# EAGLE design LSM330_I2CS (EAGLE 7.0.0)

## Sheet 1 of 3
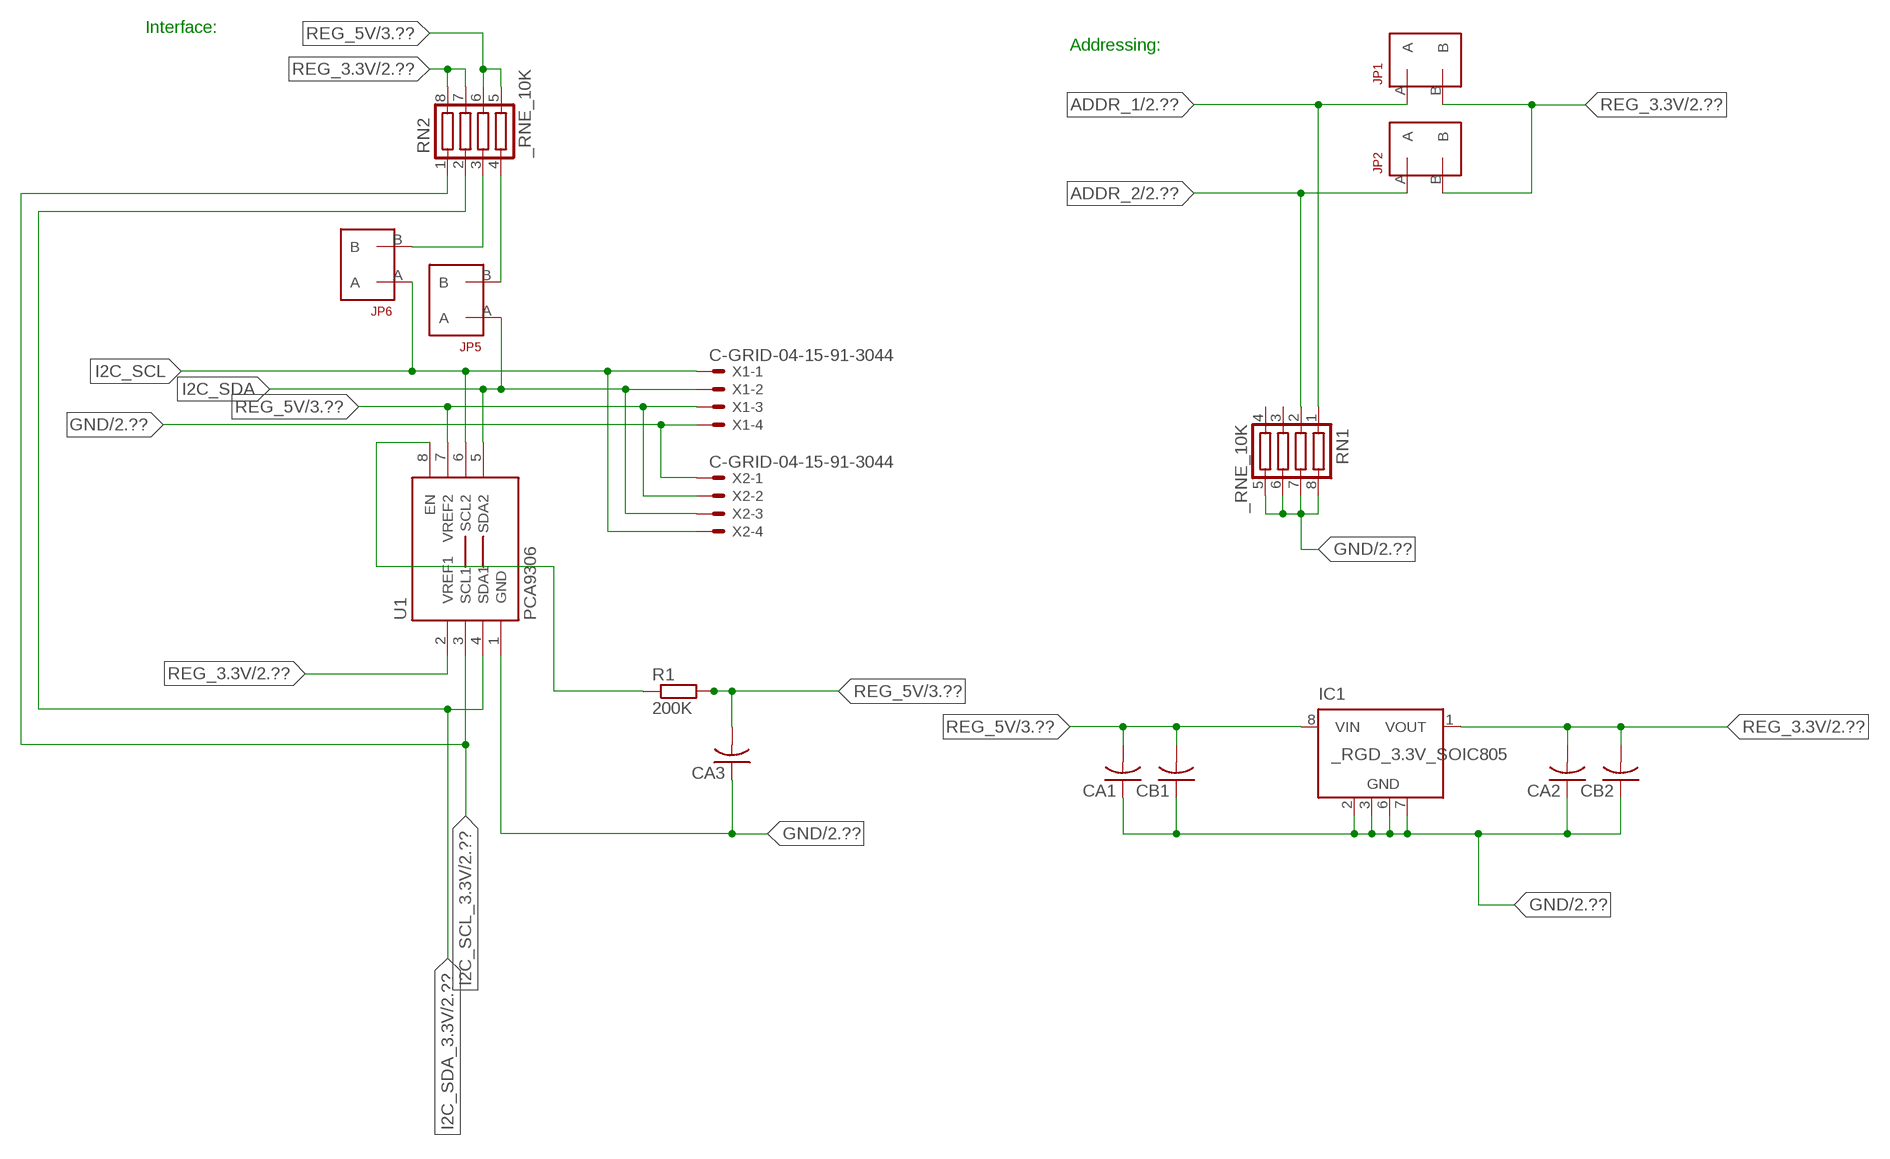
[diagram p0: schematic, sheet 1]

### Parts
CA1  CC1206KRX7R9BB104  [.1UF]
CA2  CC1206KRX7R9BB104  [.1UF]
CA3  CC1206KRX7R9BB104  [.1UF]
CB1  TMK316F106ZL-TC1206K  [TMK316F106ZL-T]
CB2  TMK316F106ZL-TC1206K  [TMK316F106ZL-T]
IC1  _RGD_3.3V_SOIC805  [_RGC_3.3V_SOIC8]
JP1  JUMPER_1X2_2MM  [JUMPER_1X2_2MM]
JP2  JUMPER_1X2_2MM  [JUMPER_1X2_2MM]
JP5  JUMPER_1X2_2MM  [JUMPER_1X2_2MM]
JP6  JUMPER_1X2_2MM  [JUMPER_1X2_2MM]
R1  200K  RESISTOR_SMT-0603  [R603]
RN1  _RNE_10K  [RNE]
RN2  _RNE_10K  [RNE]
U1  PCA9306  PCA9306_NCD  [PSOP-8]
X1  C-GRID-04-15-91-3044  [15-91-04]
X2  C-GRID-04-15-91-3044  [15-91-04]

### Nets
ADDR_1: JP1.A RN1.1 ; also sheet 2
ADDR_2: JP2.A RN1.2 ; also sheet 2
GND: CA1.1 CA2.1 CA3.1 CB1.1 CB2.1 IC1.2(GND) IC1.3(GND) IC1.6(GND) IC1.7(GND) RN1.5 RN1.6 RN1.7 RN1.8 U1.1(GND) X1.4 X2.1 ; also sheet 2,3
I2C_SCL: JP6.A U1.6(SCL2) X1.1 X2.4
I2C_SCL_3.3V: RN2.1 U1.3(SCL1) ; also sheet 2
I2C_SDA: JP5.A U1.5(SDA2) X1.2 X2.3
I2C_SDA_3.3V: RN2.2 U1.4(SDA1) ; also sheet 2
N$1: JP6.B RN2.3
N$2: JP5.B RN2.4
N$3: R1.1 U1.8(EN)
REG_3.3V: CA2.2 CB2.2 IC1.1(VOUT) JP1.B JP2.B RN2.7 RN2.8 U1.2(VREF1) ; also sheet 2
REG_5V: CA1.2 CA3.2 CB1.2 IC1.8(VIN) R1.2 RN2.5 RN2.6 U1.7(VREF2) X1.3 X2.2 ; also sheet 3
Unconnected: IC1.4(NC) IC1.5(NC) RN1.3 RN1.4

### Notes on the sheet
- Interface:
- Addressing:

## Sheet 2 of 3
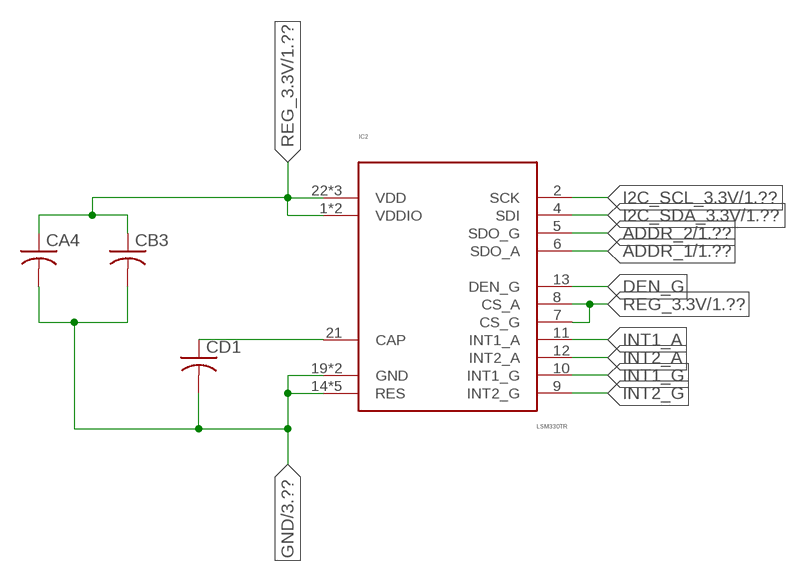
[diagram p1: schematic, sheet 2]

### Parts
CA4  CC1206KRX7R9BB104  [.1UF]
CB3  TMK316F106ZL-TC1206K  [TMK316F106ZL-T]
CD1  CC1206KRX7R9BB103C1206K  [CC1206KRX7R9BB103]
IC2  LSM330TR  LSM330  [LSM330]

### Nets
ADDR_1: IC2.6(SDO_A) ; also sheet 1
ADDR_2: IC2.5(SDO_G) ; also sheet 1
DEN_G: IC2.13(DEN_G)
GND: CA4.2 CB3.2 CD1.2 IC2.14(RES) IC2.15(RES) IC2.16(RES) IC2.17(RES) IC2.18(RES) IC2.19(GND) IC2.20(GND) ; also sheet 1,3
I2C_SCL_3.3V: IC2.2(SCK) ; also sheet 1
I2C_SDA_3.3V: IC2.4(SDI) ; also sheet 1
INT1_A: IC2.11(INT1_A)
INT1_G: IC2.10(INT1_G)
INT2_A: IC2.12(INT2_A)
INT2_G: IC2.9(INT2_G)
N$16: CD1.1 IC2.21(CAP)
REG_3.3V: CA4.1 CB3.1 IC2.1(VDDIO) IC2.3(VDDIO) IC2.7(CS_G) IC2.8(CS_A) IC2.22(VDD) IC2.23(VDD) IC2.24(VDD) ; also sheet 1

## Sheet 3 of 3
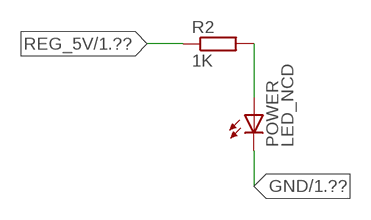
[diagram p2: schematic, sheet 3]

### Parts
POWER  LED_NCD  [CHIPLED_0603]
R2  1K  RESISTOR_SMT-0402  [R402]

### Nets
GND: POWER.C ; also sheet 1,2
N$4: POWER.A R2.2
REG_5V: R2.1 ; also sheet 1

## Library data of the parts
CA1-CA3 = NCD_ULTIMATE_LIBRARY:CC1206KRX7R9BB104: Capacitor CA .1uF 50V SMT C1206K CC1206KRX7R9BB104
CA4 = NCD_ULTIMATE_LIBRARY (2):CC1206KRX7R9BB104: Capacitor CA .1uF 50V SMT C1206K CC1206KRX7R9BB104
CB1 CB2 = NCD_ULTIMATE_LIBRARY:TMK316F106ZL-T: Capacitor CB 10uF SMT 1206 TMK316F106ZL-T
CB3 = NCD_ULTIMATE_LIBRARY (2):TMK316F106ZL-T: Capacitor CB 10uF SMT 1206 TMK316F106ZL-T
CD1 = NCD_ULTIMATE_LIBRARY (2):CC1206KRX7R9BB103: Capacitor CD .01uF SMT CC1206KRX7R9BB103 1206
IC1 = NCD_ULTIMATE_LIBRARY:_RGD_3.3V_SOIC8: Regulator Linear 3.3V Chip Positive VOLTAGE REGULATOR Digikey 497-1199-2-ND/L78L33ACD13TR
IC2 = NCD_ULTIMATE_KAMNA:LSM330
JP1 JP2 JP5 JP6 = NCD_ULTIMATE_CONNECTORS:JUMPER_1X2_2MM
POWER = NCD_ULTIMATE_LIBRARY:LED_NCD: LED Digikey 754-1132-2-ND/APT2012SRCPRV
R1 R2 = NCD_ULTIMATE_LIBRARY:RESISTOR_SMT: NCD Resistor
RN1 RN2 = NCD_ULTIMATE_LIBRARY:_RNE_10K: Resistor Array RNE SMT 10K x 4 Single Resistor Source: http://www.ctscorp.com/components/Datasheets/CTSChipArrayDs.pdf Digikey 742C083103JPTR-ND/742C083103JP; OC_FARNELL: unknown; OC_NEWARK: unknown
U1 = NCD_ULTIMATE_LIBRARY:PCA9306_NCD: NCD Bidirectional I2C level shifter. NOT compatible with all available part number pinout schemes- DOUBLE CHECK!!!; PROD_ID: IC-10023
X1 X2 = NCD_ULTIMATE_CONNECTORS:C-GRID-04: CONNECTOR 4-Pos I2C wire to board 2.54 mm (0.100") pitch header Digikey WM1342-ND/0015912045; OC_FARNELL: unknown; OC_NEWARK: unknown

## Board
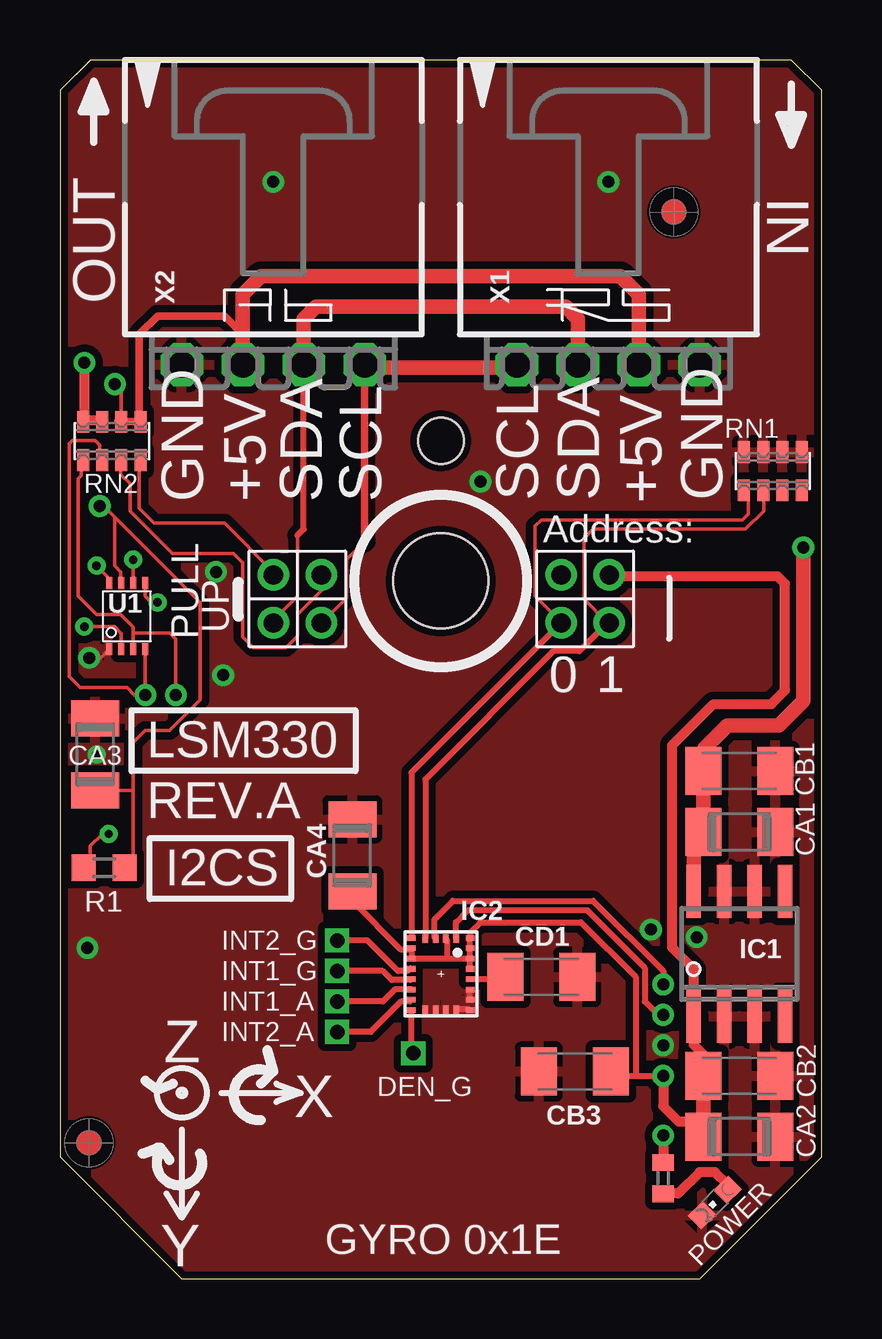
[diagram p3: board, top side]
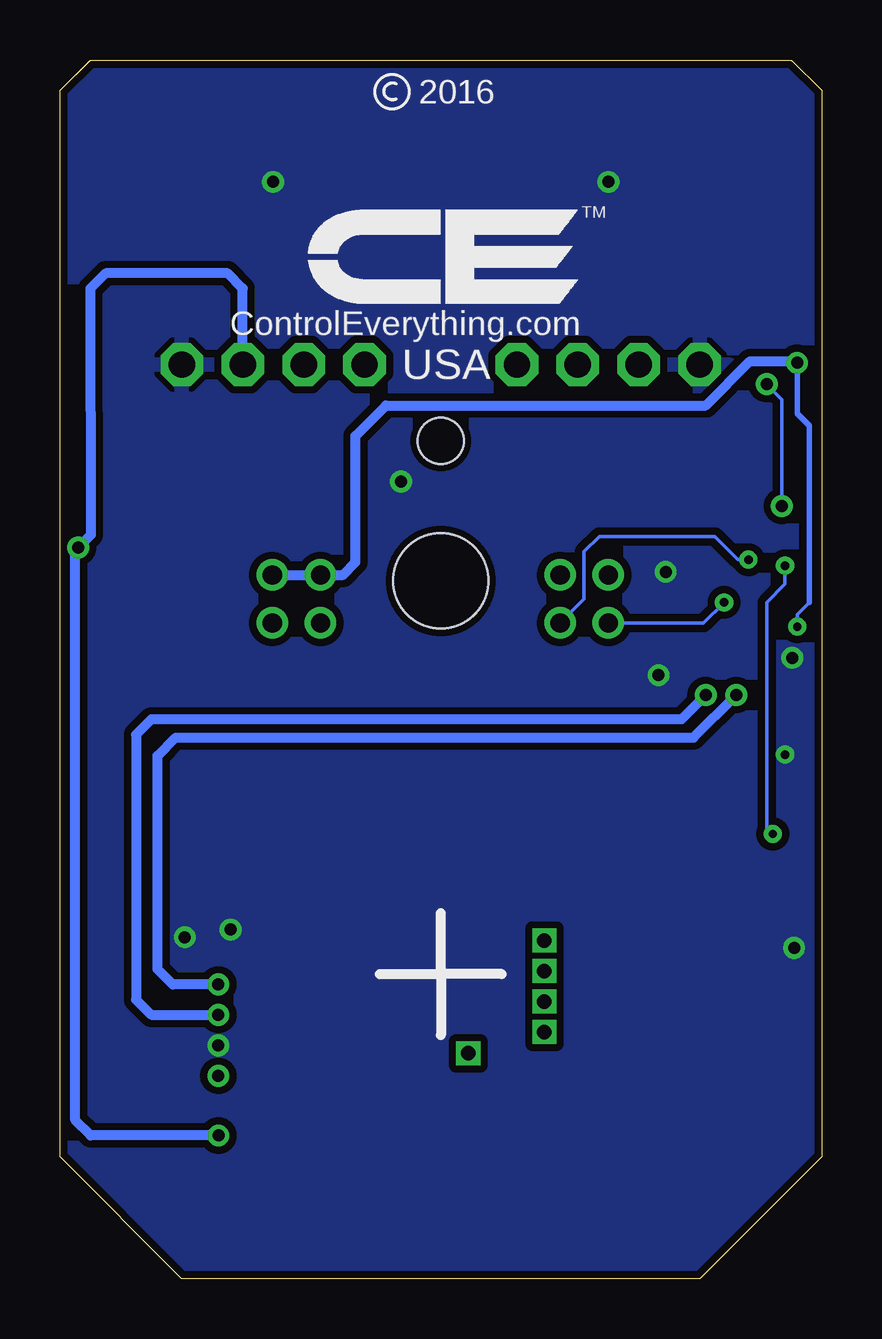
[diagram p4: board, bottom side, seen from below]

Size 31.75 x 50.8 mm. Coordinates in mm from the lower left corner, seen from the top.
Outline: 32 segments
Copper layers (1*16): Top 0.035mm / dielectric 1.5mm / Bottom 0.035mm
Design rules "default": minimum track width 5mil, minimum drill 24mil, track to track 5mil, track to pad 5mil, pad to pad 5mil, via to via 5mil, smd to smd 5mil, copper to edge 10mil, drill to drill 8mil, minimum pad ring 10mil, minimum via ring 8mil, stop-mask expansion 2mil, vias tented up to drill 0mil, thermal gap 10mil
Holes 3.96 mm at 15.88,29.08
Holes 1.91 mm at 15.88,34.93

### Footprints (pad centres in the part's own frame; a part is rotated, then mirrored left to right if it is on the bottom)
.1UF = smd 1.5 x 2: 1 -1.5,0; 2 1.5,0
TMK316F106ZL-T = smd 1.5 x 2: 1 -1.5,0; 2 1.5,0
CC1206KRX7R9BB103 = smd 1.5 x 2: 1 -1.5,0; 2 1.5,0
_RGC_3.3V_SOIC8 = smd 0.6 x 2.2: 1 -1.905,-2.6; 2 -0.635,-2.6; 3 0.635,-2.6; 4 1.905,-2.6; 5 1.905,2.6; 6 0.635,2.6; 7 -0.635,2.6; 8 -1.905,2.6
LSM330 = smd 0.23 x 0.35: 1 -1.505,1.225; 6 -1.505,-1.225; 7 -1.075,-1.225; 8 -0.645,-1.225; 9 -0.215,-1.225; 10 0.215,-1.225; 11 0.645,-1.225; 12 1.075,-1.225; 13 1.505,-1.225; 18 1.505,1.225; 19 1.075,1.225; 20 0.645,1.225; 21 0.215,1.225; 22 -0.215,1.225; 23 -0.645,1.225; 24 -1.075,1.225 | smd 0.35 x 0.23: 2 -1.475,0.645; 3 -1.475,0.215; 4 -1.475,-0.215; 5 -1.475,-0.645; 14 1.475,-0.645; 15 1.475,-0.215; 16 1.475,0.215; 17 1.475,0.645
JUMPER_1X2_2MM = drill 0.8: A 0,2; B 0,0
CHIPLED_0603 = smd 0.8 x 0.876: A 0,-0.75; C 0,0.75
R603 = smd 1 x 1.1: 1 -0.85,0; 2 0.85,0
R402 = smd 0.7 x 0.9: 1 -0.65,0; 2 0.65,0
RNE = smd 0.5 x 0.9: 1 -1.2,-0.8; 2 -0.4,-0.8; 3 0.4,-0.8; 4 1.2,-0.8; 5 1.2,0.8; 6 0.4,0.8; 7 -0.4,0.8; 8 -1.2,0.8
PSOP-8 = smd 0.25 x 0.5: 1 -0.73,-1.37; 2 -0.23,-1.37; 3 0.27,-1.37; 4 0.77,-1.37; 5 0.77,1.38; 6 0.27,1.38; 7 -0.23,1.38; 8 -0.73,1.38
15-91-04 = drill 1.1 pad 1.778 octagon: 1 -3.81,-7.62; 2 -1.27,-7.62; 3 1.27,-7.62; 4 3.81,-7.62

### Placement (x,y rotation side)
CA1  28.32,18.62 180 top
CA2  28.32,5.92 180 top
CA3  1.46,21.86 270 top
CA4  12.19,17.65 90 top
CB1  28.32,21.16 180 top
CB2  28.32,8.46 180 top
CB3  21.46,8.64 180 top
CD1  20.07,12.57 0 top
IC1  28.32,13.54 0 top
IC2  15.88,12.7 270 top
JP1  20.89,29.34 180 top
JP2  22.9,29.34 180 top
JP5  8.89,29.34 180 top
JP6  10.9,29.34 180 top
POWER  27.3,3.18 135 top
R1  1.84,17.13 0 top
R2  25.15,4.19 270 top
RN1  29.72,33.66 0 top
RN2  2.16,34.93 0 top
U1  2.79,27.61 0 top
U$5  [VISION_REF10]  1.21,5.66 90 top
U$28  [VISION_REF10]  25.59,44.46 90 top
X1  22.86,45.72 0 top
X2  8.89,45.72 0 top

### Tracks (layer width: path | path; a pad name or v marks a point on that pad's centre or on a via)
ADDR_1
  Top 0.152: JP1.A 20.89,27.37 19.81,28.45 19.81,31.37 20.07,31.62 28.45,31.62 28.7,31.88 28.7,32.78 RN1.1
  Top 0.254: JP1.A 14.65,21.09 IC2.6
ADDR_2
  Top 0.152: JP2.A 22.83,27.34 21.84,28.32 21.84,30.86 22.23,31.24 28.57,31.24 29.34,32 29.34,32.59 RN1.2
  Top 0.254: 22.83,27.34 21.65,26.16 20.57,26.16 15.23,20.82 IC2.5
DEN_G  (via drill 0.6)
  Top 0.254: v14.73,9.4 14.65,9.48 IC2.13
GND  (via drill 0.35, 0.5)
  Top 0.152: CA3.1 1.52,23.42 1.52,23.62 | U1.1 1.7,25.88 v1.22,25.88
  Top 0.254: IC2.18 17.07,11.23 IC2.17 | IC2.19 IC2.20
  other vias: 8.89,45.72 22.86,45.72 25.15,9.73 6.8,25.16 17.53,33.22 26.55,14.24 1.15,13.79 6.5,29.46 1.52,21.84 24.64,14.55
  pour Top (isolate 0.305): -1.27,0 -1.27,50.8 33.02,50.8 33.02,0
  pour Bottom (isolate 0.305): -5.08,0 -5.08,50.8 35.56,50.8 35.56,0
I2C_SCL  (via drill 0.35)
  Top 0.152: 12.7,30.73 11.94,29.97 11.94,28.38 JP6.A | v3.05,29.97 3.06,29.96 U1.6
  Top 0.305: 12.7,30.73 X2.4
  Top 0.406: X2.4 12.7,37.97 | 19.05,37.97 X1.1
  Top 0.61: 12.7,37.97 19.05,37.97
  Bottom 0.152: JP6.A 9.91,28.33 9.91,30.3 9.27,30.94 4.45,30.94 3.48,29.97 v3.05,29.97
I2C_SCL_3.3V  (via drill 0.5)
  Top 0.152: RN2.1 0.89,34.07 0.89,33.48 0.77,33.35 0.77,29.1 0.76,29.09 0.76,28.45 1.52,27.69 2.54,27.69 3.06,27.17 3.06,26.92 | 3.06,26.92 U1.3 | v4.83,24.33 v4.83,24.34 4.83,26.67 4.57,26.92 3.06,26.92
  Top 0.254: IC2.2 16.51,14.19 16.51,14.86 17.02,15.37 21.97,15.37 24.38,12.95 24.38,11.56 24.94,11 v25.15,11
  Bottom 0.406: v4.83,24.33 5.84,23.32 27.94,23.32 28.58,22.68 28.58,11.63 27.94,11 v25.15,11
I2C_SDA  (via drill 0.35)
  Top 0.152: JP5.A 8.89,27.44 9.91,28.45 9.91,30.99 | U1.5 3.56,28.45 3.81,28.19 v4.06,28.19
  Top 0.254: 9.91,30.99 10.16,31.25 X2.3
  Top 0.61: X2.3 10.16,40.01 10.67,40.51 21.09,40.51 21.59,40.01 X1.2
  Bottom 0.152: v4.06,28.19 4.92,27.34 JP5.A
I2C_SDA_3.3V  (via drill 0.5)
  Top 0.152: RN2.2 1.65,34.14 1.65,34.75 1.46,34.94 0.51,34.94 0.38,34.81 0.38,26.37 0.38,26.36 0.38,25.1 0.84,24.64 2.79,24.64 3.1,24.33 v3.56,24.33 v3.56,24.34 U1.4
  Top 0.254: 25.15,12.44 v25.15,12.27 25.15,12.82 22.23,15.75 16.38,15.75 15.62,14.99 15.62,14.21 IC2.4
  Bottom 0.406: v25.15,12.27 27.05,12.27 27.69,12.9 27.69,21.79 26.93,22.56 5.34,22.56 v3.56,24.33
INT1_A  (via drill 0.6)
  Top 0.254: IC2.11 14.64,12.07 13.97,12.07 13.46,11.56 v11.56,11.56
INT1_G  (via drill 0.6)
  Top 0.254: IC2.10 14.61,12.45 13.84,12.45 13.46,12.83 v11.56,12.83
INT2_A  (via drill 0.6)
  Top 0.254: IC2.12 14.58,11.56 14.22,11.56 12.95,10.29 v11.56,10.29
INT2_G  (via drill 0.6)
  Top 0.254: IC2.9 14.61,12.95 14.48,12.83 14.1,12.83 12.83,14.1 v11.56,14.1
N$1
  Top 0.152: JP6.B 10.92,29.31 10.92,28.7 9.91,27.69 9.91,26.8 9.42,26.31 8.06,26.31 7.62,26.75 7.62,29.84 7.24,30.23 4.7,30.23 2.92,32 2.92,33.15 2.54,33.53 2.54,34.1 RN2.3
  Top 0.305: 2.54,34.02 RN2.3
N$2
  Top 0.152: JP5.B 8.89,29.46 6.86,31.5 3.94,31.5 3.3,32.13 3.3,34.07 RN2.4
  Top 0.305: 3.37,33.88 RN2.4
N$3  (via drill 0.35)
  Top 0.152: R1.1 1.27,17.41 1.27,18.03 1.78,18.54 v2.03,18.54 | v1.52,29.72 2.06,29.18 U1.8
  Bottom 0.152: v2.03,18.54 2.29,18.8 2.29,28.19 1.52,28.96 v1.52,29.72
N$4
  Top 0.406: POWER.A 27.84,3.92 27.3,4.45 26.67,4.45 25.78,3.56 25.16,3.56 R2.2
N$16
  Top 0.254: CD1.1 18.48,12.49 IC2.21
REG_3.3V  (via drill 0.35, 0.5)
  Top 0.152: v1.02,27.18 2.29,27.18 2.56,26.9 U1.2
  Top 0.254: IC2.22 IC2.23 | IC2.23 IC2.24 IC2.1 17.1,14.43 17.53,14.86 21.72,14.86 24,12.57 24,8.46 | 16.13,13.35 IC2.8 IC2.7 14.59,13.72 14.22,13.72 12.19,15.75 CA4.1 | 16.13,13.35 IC2.23 | IC2.3 16.13,14.14 16.13,13.35 | CB3.1 23.14,8.46 24,8.46 | 24,8.46 v25.15,8.46
  Top 0.406: CB2.2 26.82,9.35 26.42,9.75 26.42,10.36 | v25.15,8.46 25.15,7.19 25.78,6.55 26.82,6.55 | IC1.1 26.42,12.9 25.53,13.79 25.53,22.24 27.24,23.95 29.66,23.95 30.23,24.52 30.23,28.97 29.91,29.29 22.95,29.29 JP2.B | 26.52,5.62 CA2.2 | v1.02,38.18 1.02,35.78 | 1.02,35.78 RN2.8 | 1.02,35.78 1.71,35.78 RN2.7
  Top 0.61: CB2.2 26.82,6.55 CA2.2 | 26.42,10.36 IC1.1
  Bottom 0.152: 0.51,28.19 1.02,27.69 v1.02,27.18
  Bottom 0.229: 0.51,28.19 0.51,35.56 1.02,36.07 v1.02,38.18
  Bottom 0.406: v1.02,38.18 1.08,38.24 2.99,38.24 4.83,36.4 18.16,36.4 19.43,35.13 19.43,29.87 19.94,29.34 JP1.B JP2.B
REG_5V  (via drill 0.5)
  Top 0.152: RN2.6 2.56,37.01 v2.29,37.29 | R1.2 3.05,17.49 3.05,20.36 | 3.05,20.36 3.05,22.35 3.56,22.86 4.57,22.86 5.84,24.13 5.84,28.19 2.29,31.75 | CA3.2 3.05,20.36 | 2.29,31.75 1.83,32.21 v1.65,32.21 | U1.7 2.54,29.01 2.54,29.46 2.29,29.72 2.29,31.75
  Top 0.305: 7.62,39.37 7.5,39.37 | 2.42,35.74 RN2.6 RN2.5 3.31,35.8 3.31,39.37 4.07,40.13 6.86,40.13 7.62,39.37 | X2.2 7.62,39.37
  Top 0.406: v25.15,5.97 R2.1
  Top 0.61: X2.2 7.62,41.02 8.38,41.78 23.37,41.78 24.13,41.02 X1.3 | IC1.8 26.42,18.21 CA1.2 CB1.2 26.86,21.2 26.86,22.11 27.82,23.06 29.98,23.06 30.99,24.08 v30.99,30.48
  Bottom 0.152: v1.65,32.21 1.65,36.65 v2.29,37.29
  Bottom 0.406: X1.3 24.13,41.28 24.77,41.91 29.84,41.91 30.48,41.27 30.47,31 v30.99,30.48 31.11,30.36 31.11,6.6 30.48,5.97 v25.15,5.97

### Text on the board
tNames: IN | OUT | GND | +5V | SDA | SCL | SCL | SDA | +5V | GND | Address: | PULL | UP | 0 | 1 | LSM330 | REV.A | I2CS | INT2_G | INT1_G | INT1_A | INT2_A | Z | DEN_G | X | Y | GYRO 0x1E
bNames: 2016 | TM | ControlEverything.com | USA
